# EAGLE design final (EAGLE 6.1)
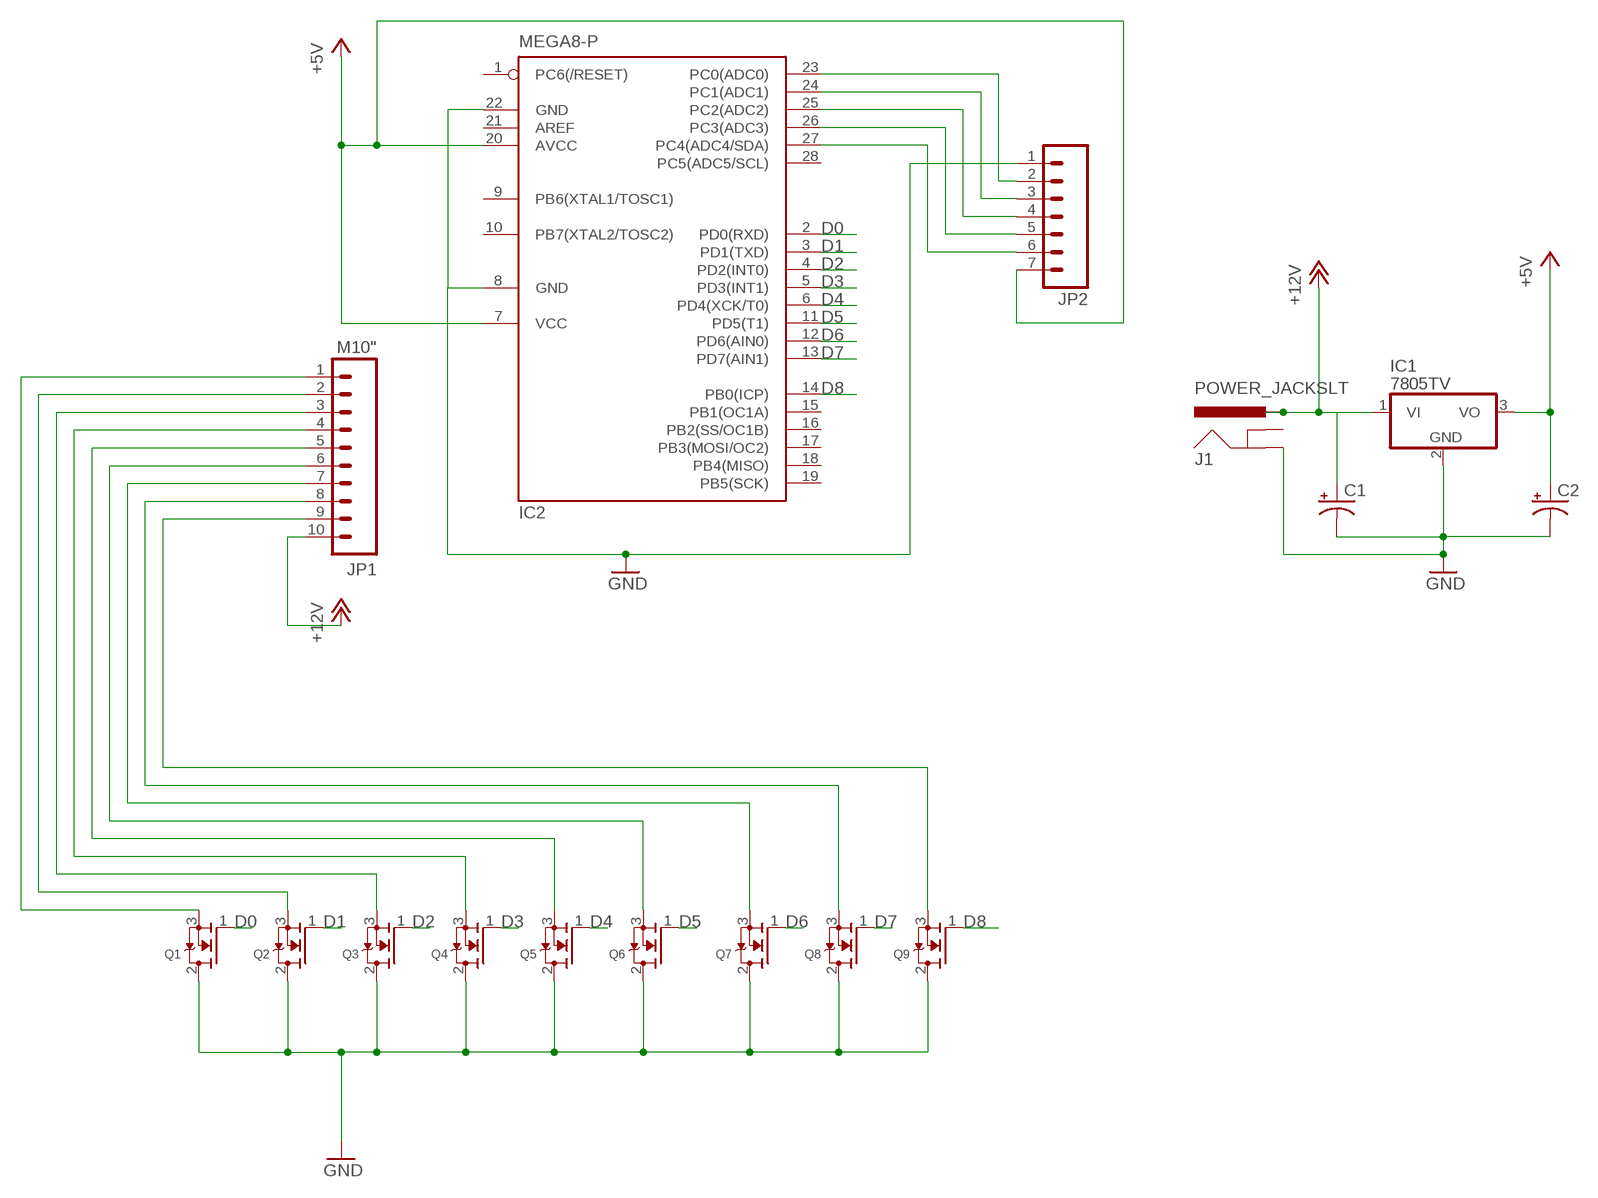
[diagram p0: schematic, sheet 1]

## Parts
C1  CAP_POLPTH1  [CPOL-RADIAL-100UF-25V]
C2  CAP_POLPTH1  [CPOL-RADIAL-100UF-25V]
IC1  7805TV  [TO220V]
IC2  MEGA8-P  [DIL28-3]
J1  POWER_JACKSLT  [POWER_JACK_SLOT]
JP1  M10"  [1X10]
JP2  M07  [1X07]
Q1  MOSFET-NGDS_TO220V  [TO220V]
Q2  MOSFET-NGDS_TO220V  [TO220V]
Q3  MOSFET-NGDS_TO220V  [TO220V]
Q4  MOSFET-NGDS_TO220V  [TO220V]
Q5  MOSFET-NGDS_TO220V  [TO220V]
Q6  MOSFET-NGDS_TO220V  [TO220V]
Q7  MOSFET-NGDS_TO220V  [TO220V]
Q8  MOSFET-NGDS_TO220V  [TO220V]
Q9  MOSFET-NGDS_TO220V  [TO220V]

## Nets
+5V: C2.1(+) IC1.3(VO) IC2.7(VCC) IC2.20(AVCC) JP2.7
+12V: C1.1(+) IC1.1(VI) J1.PWR JP1.10
D0: IC2.2(PD0(RXD)) Q1.1(G)
D1: IC2.3(PD1(TXD)) Q2.1(G)
D2: IC2.4(PD2(INT0)) Q3.1(G)
D3: IC2.5(PD3(INT1)) Q4.1(G)
D4: IC2.6(PD4(XCK/T0)) Q5.1(G)
D5: IC2.11(PD5(T1)) Q6.1(G)
D6: IC2.12(PD6(AIN0)) Q7.1(G)
D7: IC2.13(PD7(AIN1)) Q8.1(G)
D8: IC2.14(PB0(ICP)) Q9.1(G)
GND: C1.2(-) C2.2(-) IC1.2(GND) IC2.8(GND) IC2.22(GND) J1.GND@2(GND) JP2.1 Q1.2(D) Q2.2(D) Q3.2(D) Q4.2(D) Q5.2(D) Q6.2(D) Q7.2(D) Q8.2(D) Q9.2(D)
N$1: JP1.1 Q1.3(S)
N$2: JP1.2 Q2.3(S)
N$3: JP1.3 Q3.3(S)
N$4: IC2.27(PC4(ADC4/SDA)) JP2.6
N$5: IC2.23(PC0(ADC0)) JP2.2
N$6: IC2.24(PC1(ADC1)) JP2.3
N$7: IC2.25(PC2(ADC2)) JP2.4
N$8: IC2.26(PC3(ADC3)) JP2.5
N$9: JP1.4 Q4.3(S)
N$10: JP1.5 Q5.3(S)
N$11: JP1.6 Q6.3(S)
N$12: JP1.7 Q7.3(S)
N$13: JP1.8 Q8.3(S)
N$14: JP1.9 Q9.3(S)
Unconnected: IC2.1(PC6(/RESET)) IC2.9(PB6(XTAL1/TOSC1)) IC2.10(PB7(XTAL2/TOSC2)) IC2.15(PB1(OC1A)) IC2.16(PB2(SS/OC1B)) IC2.17(PB3(MOSI/OC2)) IC2.18(PB4(MISO)) IC2.19(PB5(SCK)) IC2.21(AREF) IC2.28(PC5(ADC5/SCL)) J1.GND@1(GNDBREAK)

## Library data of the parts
C1 C2 = SparkFun:CAP_POL: Capacitor Polarized
IC1 = linear:78*: Positive VOLTAGE REGULATOR Source: http://cache.national.com/ds/LM/LM78L05.pdf http://www.fairchildsemi.com/ds/LM/LM7805.pdf
IC2 = atmel:MEGA8-P: MICROCONTROLLER 8 Kbytes FLASH, 1 kbytes SRAM, 512 bytes EEPROM, USART, 4-channel 10 bit ADC, 2-channel 8 bit ADC Pin compatible with Atmega48, ATMega88, ATMega168 Source: avr.lbr; OC_FARNELL: unknown; OC_NEWARK: unknown
J1 = SparkFun:POWER_JACK: Power Jack This is the standard 5.5mm barrel jack for power. The PTH is the most common, proven, reliable, footprint. All others are experimental. The Slot footprint only works if the mill layer is transmitted to the PCB fab house so be warned. Spark Fun Electronics SKU : PRT-00119. Mating wall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
JP1 = SparkFun:M10: Header 10 Standard 10-pin 0.1" header. Use with straight break away headers (SKU : PRT-00116), right angle break away headers (PRT-00553), swiss pins (PRT-00743), machine pins (PRT-00117), and female headers (PRT-00115).
JP2 = SparkFun:M07: Header 7 Standard 7-pin 0.1" header. Use with straight break away headers (SKU : PRT-00116), right angle break away headers (PRT-00553), swiss pins (PRT-00743), machine pins (PRT-00117), and female headers (PRT-00115). NOTES ON THE VARIANTS LOCK and LOCK_LONGPADS... This footprint was designed to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
Q1-Q9 = adafruit:MOSFET-N: N-Channel Mosfet 2N7002E - 60V 260mA SOT23 [Digikey: 2N7002ET1GOSTR-ND] - REEL BSH103 - 30V 850mA SOT23 [Digikey: 568-5013-1-ND]

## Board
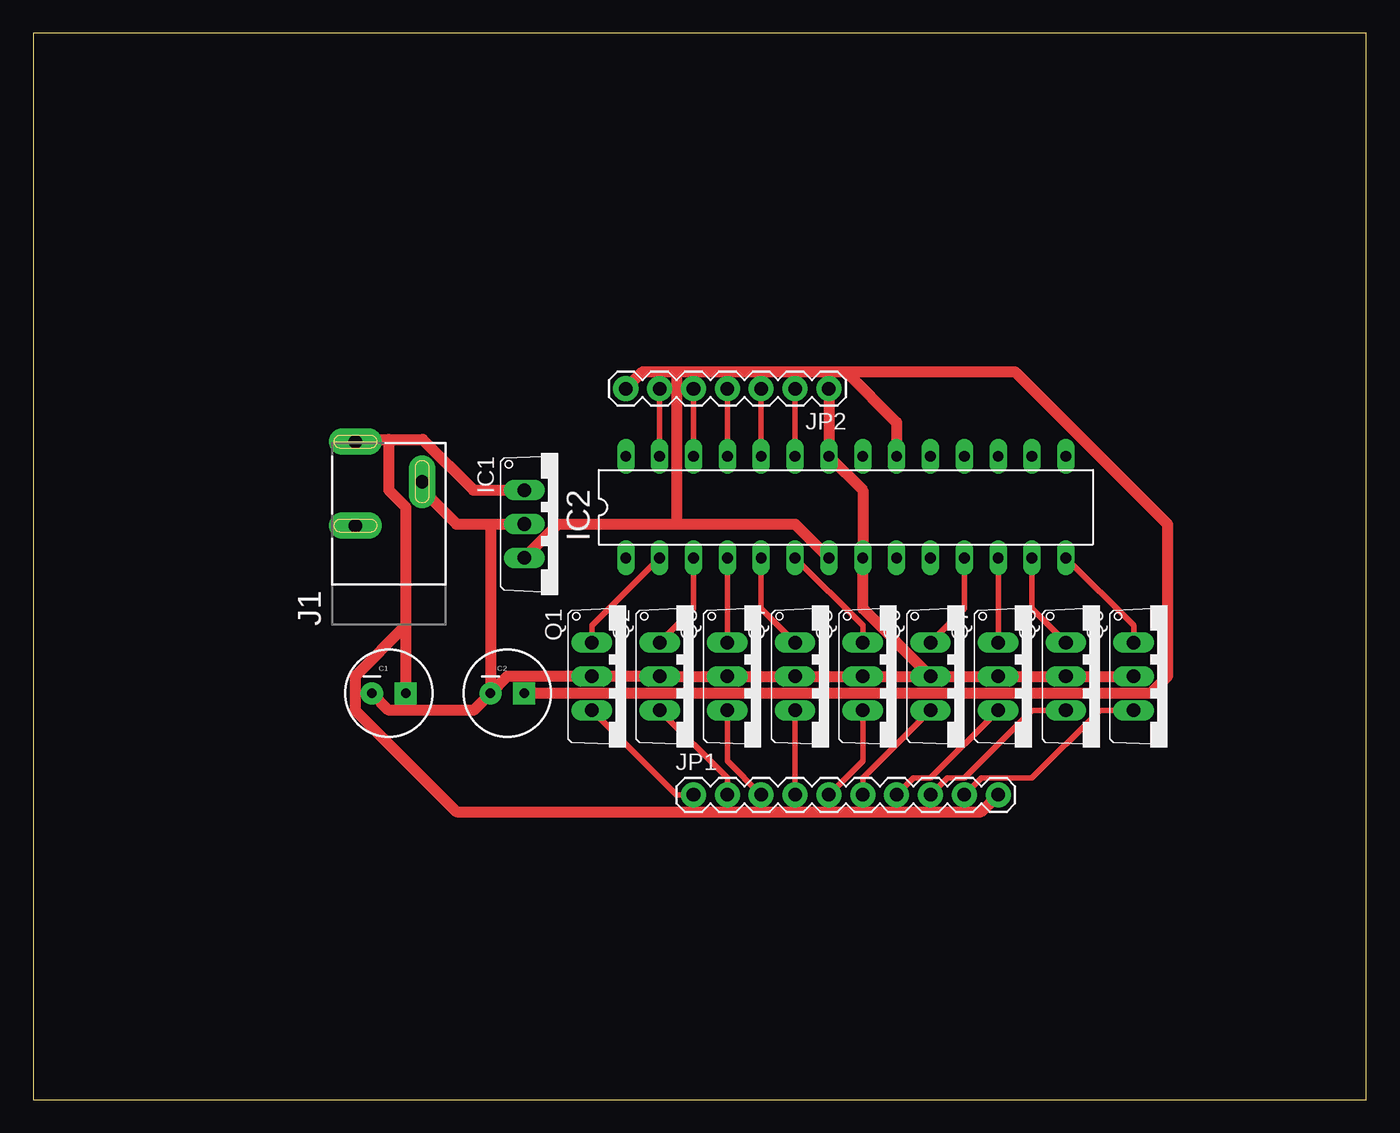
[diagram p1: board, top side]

Size 100 x 80 mm. Coordinates in mm from the lower left corner, seen from the top.
Outline: 0,0 100,0 100,80 0,80 0,0
Copper layers (1*16): Top 0.035mm / dielectric 1.5mm / Bottom 0.035mm
Design rules: minimum track width 10mil, minimum drill 24mil, track to track 8mil, track to pad 8mil, pad to pad 8mil, via to via 8mil, smd to smd 8mil, copper to edge 40mil, drill to drill 8mil, minimum pad ring 10mil, minimum via ring 8mil, stop-mask expansion 4mil, vias tented up to drill 0mil, thermal gap 10mil

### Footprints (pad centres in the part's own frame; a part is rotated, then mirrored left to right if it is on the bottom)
CPOL-RADIAL-100UF-25V = drill 0.7 pad 1.651 square: 1 1.27,0 | drill 0.7 pad 1.651: 2 -1.27,0
TO220V = drill 1.016 long: 1 -2.54,-2.54; 2 0,-2.54; 3 2.54,-2.54
DIL28-3 = drill 0.813 long: 1 -16.51,-3.81; 2 -13.97,-3.81; 3 -11.43,-3.81; 4 -8.89,-3.81; 5 -6.35,-3.81; 6 -3.81,-3.81; 7 -1.27,-3.81; 8 1.27,-3.81; 9 3.81,-3.81; 10 6.35,-3.81; 11 8.89,-3.81; 12 11.43,-3.81; 13 13.97,-3.81; 14 16.51,-3.81; 15 16.51,3.81; 16 13.97,3.81; 17 11.43,3.81; 18 8.89,3.81; 19 6.35,3.81; 20 3.81,3.81; 21 1.27,3.81; 22 -1.27,3.81; 23 -3.81,3.81; 24 -6.35,3.81; 25 -8.89,3.81; 26 -11.43,3.81; 27 -13.97,3.81; 28 -16.51,3.81
POWER_JACK_SLOT = drill 1 pad 2 long: GND@1 2.58,7.5; GND@2 7.58,10.8; PWR 2.58,13.8
1X10 = drill 1.016 pad 1.88: 1 0,0; 2 2.54,0; 3 5.08,0; 4 7.62,0; 5 10.16,0; 6 12.7,0; 7 15.24,0; 8 17.78,0; 9 20.32,0; 10 22.86,0
1X07 = drill 1.016 pad 1.88: 1 0,0; 2 2.54,0; 3 5.08,0; 4 7.62,0; 5 10.16,0; 6 12.7,0; 7 15.24,0

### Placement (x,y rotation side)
C1  26.67,30.48 0 top
C2  35.56,30.48 0 top
IC1  39.37,43.18 270 top
IC2  60.96,44.45 0 top
J1  21.59,35.56 0 top
JP1  49.53,22.86 0 top
JP2  59.69,53.34 180 top
Q1  44.45,31.75 270 top
Q2  49.53,31.75 270 top
Q3  54.61,31.75 270 top
Q4  59.69,31.75 270 top
Q5  64.77,31.75 270 top
Q6  69.85,31.75 270 top
Q7  74.93,31.75 270 top
Q8  80.01,31.75 270 top
Q9  85.09,31.75 270 top

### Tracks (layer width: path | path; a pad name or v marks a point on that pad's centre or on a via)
+5V
  Top 0.813: IC2.7 57.15,43.18 48.26,43.18 | 48.26,43.18 39.37,43.18 IC1.3 | IC2.20 64.77,50.8 60.96,54.61 | 48.26,54.61 45.72,54.61 JP2.7 | 48.26,54.61 60.96,54.61 | C2.1 83.82,30.48 85.09,31.75 85.09,43.18 73.66,54.61 60.96,54.61 | 48.26,54.61 48.26,43.18
+12V
  Top 0.813: IC1.1 33.02,45.72 29.21,49.53 26.67,49.53 | 26.67,49.53 25.4,49.53 J1.PWR | 27.94,35.56 27.94,44.45 26.67,45.72 26.67,49.53 | 27.94,35.56 C1.1 | JP1.10 71.12,21.59 31.75,21.59 24.13,29.21 24.13,31.75 27.94,35.56
D0
  Top 0.406: IC2.2 41.91,35.56 Q1.1
D1
  Top 0.406: IC2.3 49.53,36.83 Q2.1
D2
  Top 0.406: Q3.1 IC2.4
D3
  Top 0.406: IC2.5 54.61,36.83 Q4.1
D4
  Top 0.406: IC2.6 62.23,35.56 Q5.1
D5
  Top 0.406: IC2.11 69.85,36.83 Q6.1
D6
  Top 0.406: Q7.1 IC2.12
D7
  Top 0.406: IC2.13 74.93,36.83 Q8.1
D8
  Top 0.406: IC2.14 82.55,35.56 Q9.1
GND
  Top 0.813: C1.2 26.67,29.21 33.02,29.21 C2.2 | 34.29,43.18 31.75,43.18 29.21,45.72 J1.GND@2 | 34.29,43.18 IC1.2 | 34.29,43.18 C2.2 | JP2.1 IC2.22 62.23,45.72 IC2.8 62.23,36.83 Q6.2 | Q6.2 Q5.2 Q4.2 Q3.2 Q2.2 Q1.2 35.56,31.75 C2.2 | Q6.2 Q7.2 Q8.2 Q9.2
N$1
  Top 0.406: Q1.3 48.26,22.86 JP1.1
N$2
  Top 0.406: Q2.3 52.07,24.13 JP1.2
N$3
  Top 0.406: Q3.3 52.07,25.4 JP1.3
N$4
  Top 0.406: JP2.6 IC2.27
N$5
  Top 0.406: JP2.2 IC2.23
N$6
  Top 0.406: JP2.3 IC2.24
N$7
  Top 0.406: JP2.4 IC2.25
N$8
  Top 0.406: JP2.5 IC2.26
N$9
  Top 0.406: JP1.4 Q4.3
N$10
  Top 0.406: Q5.3 62.23,25.4 JP1.5
N$11
  Top 0.406: Q6.3 62.23,24.13 JP1.6
N$12
  Top 0.406: Q7.3 67.31,24.13 66.04,24.13 JP1.7
N$13
  Top 0.406: Q8.3 74.93,29.21 69.85,24.13 68.58,24.13 JP1.8
N$14
  Top 0.406: Q9.3 80.01,29.21 74.93,24.13 71.12,24.13 JP1.9

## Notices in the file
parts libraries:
SparkFun: Licensing: CC v3.0 Share-Alike You are welcome to use this library for commercial purposes.
